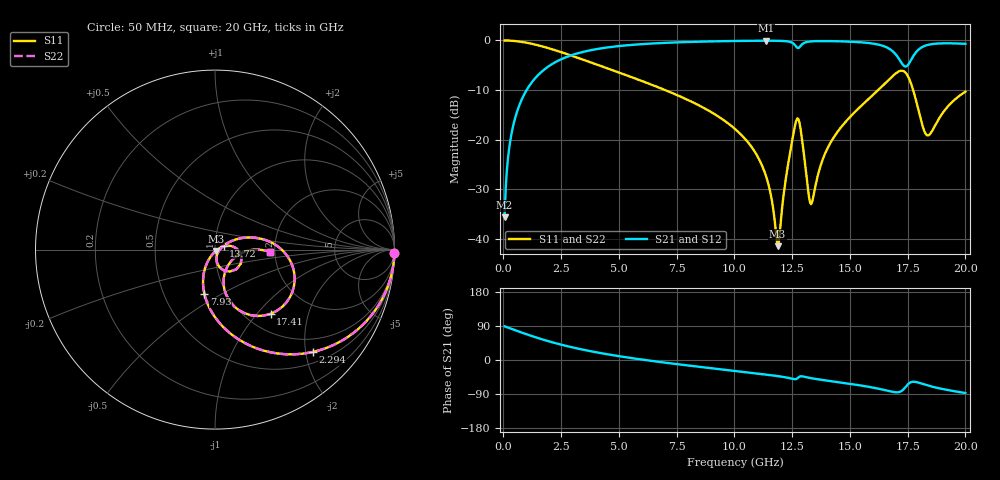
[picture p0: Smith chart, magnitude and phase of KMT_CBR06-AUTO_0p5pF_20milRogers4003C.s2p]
! Data measured by Modelithics Inc. support@modelithics.com 813-866-6335
! KEMET CBR06-AUTO 0.5pF, Pad Width= 0.851mm, Pad Length= 0.64mm, Pad Gap= 0.62mm, 20mil Rogers 4003C substrate Data, January 2022
# hz S ma R 50
! 2 Port Network Data from SP1.SP block
! freq  magS11  angS11  magS21  angS21  magS12  angS12  magS22  angS22
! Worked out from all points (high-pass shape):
!   401 points, 50 MHz to 20 GHz, reference 50 ohm
!   highest |S21| = -0.06 dB at 11.37 GHz (marker M1); lowest = -35.6 dB at 50 MHz (marker M2)
!   |S21| within 3 dB of the highest: 2.897 GHz to 17.03 GHz (14.13 GHz wide, 142 % of centre); 17.76 GHz to end of sweep
!   lowest |S11| = -41.5 dB at 11.87 GHz (marker M3), VSWR 1.02, Z = 50.4 - j0.73 ohm
!   |S11| at or under -10 dB: 6.996 GHz to 16.22 GHz (9.228 GHz wide, 79.5 % of centre); 17.74 GHz to end of sweep
!   |S22| runs from -41.5 to 0.0 dB; largest |S21 - S12| = 0
!   S11 on the Smith chart (normalised r, x): 50 MHz: open; 2.294 GHz: 0.71, -2.15; 7.93 GHz: 0.79, -0.42; 13.72 GHz: 1.10, +0.05; 17.41 GHz: 1.29, -1.19; 20 GHz: 1.87, -0.05
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5e7  0.9999 -1.1  0.01655 88.9  0.01655 88.9  0.9999 -1.1
2.99375e8  0.9951 -6.8  0.09868 83.2  0.09868 83.2  0.9951 -6.8
6.485e8  0.9775 -14.5  0.2102 75.5  0.2102 75.5  0.9775 -14.5
2.294375e9  0.7896 -46.2  0.6122 43.7  0.6122 43.7  0.7896 -46.2
3.391625e9  0.6468 -62.0  0.7608 27.9  0.7608 27.9  0.6468 -62.0
6.73325e9  0.3346 -94.5  0.9395 -5.0  0.9395 -5.0  0.3346 -94.5
7.93025e9  0.2546 -103.4  0.9639 -14.0  0.9639 -14.0  0.2546 -103.4
1.0025e10  0.1282 -117.2  0.9878 -28.8  0.9878 -28.8  0.1282 -117.2
1.137162e10  0.04262 -121.3  0.9935 -38.4  0.9935 -38.4  0.04262 -121.3
1.187038e10  0.008431 -59.1  0.9915 -42.4  0.9915 -42.4  0.008431 -59.1
1.236912e10  0.06516 18.6  0.9715 -47.7  0.9715 -47.7  0.06516 18.6
1.271825e10  0.1638 -28.4  0.8444 -48.7  0.8444 -48.7  0.1638 -28.4
1.286788e10  0.1266 -66.8  0.8824 -43.0  0.8824 -43.0  0.1266 -66.8
1.3217e10  0.02767 -61.5  0.9728 -46.8  0.9728 -46.8  0.02767 -61.5
1.336662e10  0.02359 -12.8  0.9803 -48.5  0.9803 -48.5  0.02359 -12.8
1.371575e10  0.05335 24.4  0.9855 -51.8  0.9855 -51.8  0.05335 24.4
1.46135e10  0.133 25.6  0.9794 -59.5  0.9794 -59.5  0.133 25.6
1.670825e10  0.4067 -5.5  0.824 -82.2  0.824 -82.2  0.4067 -5.5
1.74065e10  0.4735 -49.0  0.5455 -71.6  0.5455 -71.6  0.4735 -49.0
1.78055e10  0.2786 -75.3  0.7305 -57.5  0.7305 -57.5  0.2786 -75.3
1.835412e10  0.1103 -40.7  0.8993 -67.0  0.8993 -67.0  0.1103 -40.7
2e10  0.3044 -2.3  0.9247 -87.2  0.9247 -87.2  0.3044 -2.3
